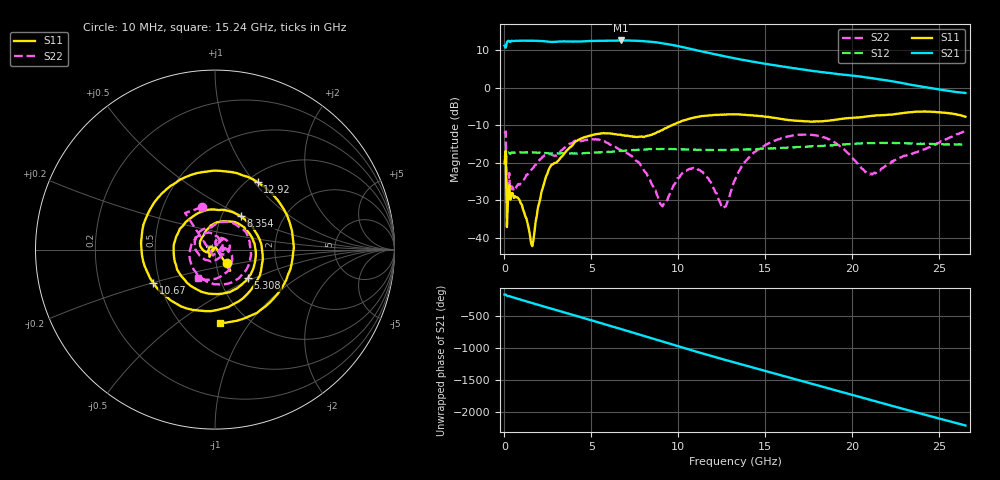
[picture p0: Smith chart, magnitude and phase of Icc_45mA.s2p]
!Keysight Technologies,N5245A,MY52451697,A.10.60.06
!Date: Thursday, May 06, 2021 15:05:53
!Correction: S11(Full 2 Port(1,4))
!S41(Full 2 Port(1,4))
!S14(Full 2 Port(1,4))
!S44(Full 2 Port(1,4))
!S2P File: Measurements: S11, S41, S14, S44:
# Hz S  dB  R 50
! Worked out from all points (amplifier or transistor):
!   401 points, 10 MHz to 26.5 GHz, reference 50 ohm
!   highest |S21| = 12.7 dB at 6.699 GHz (marker M1)
!   |S21| within 3 dB of that: start of sweep to 11.42 GHz
!   unconditionally stable (mu >= 1): start of sweep to end of sweep
!   at 4.381 GHz: K = 1.13, MAG = 12.7 dB, |S12| = -17.4 dB
!   at 13.26 GHz: K = 1.24, MAG = 9.2 dB, |S12| = -16.5 dB
!   at 26.5 GHz: K = 2.53, MAG = 0.0 dB, |S12| = -15.0 dB
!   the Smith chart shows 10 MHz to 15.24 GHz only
!   S11 on the Smith chart (normalised r, x): 10 MHz: 1.13, -0.17; 5.308 GHz: 1.37, -0.46; 8.354 GHz: 1.23, +0.48; 10.67 GHz: 0.46, -0.20; 12.92 GHz: 1.11, +1.04; 15.24 GHz: 0.75, -0.73
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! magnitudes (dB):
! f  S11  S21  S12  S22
! 10 MHz  -20.1  11.3  -18.0  -12.1
! 274.9 MHz  -25.9  12.5  -17.4  -22.7
! 870.9 MHz  -29.9  12.6  -17.2  -25.8
! 1.599 GHz  -42.2  12.6  -17.2  -21.6
! 2.063 GHz  -29.4  12.5  -17.2  -18.9
! 2.593 GHz  -21.3  12.3  -17.5  -17.6
! 4.447 GHz  -13.4  12.4  -17.4  -14.1
! 5.308 GHz  -12.3  12.6  -17.2  -13.7
! 6.699 GHz  -12.5  12.7  -16.8  -16.6
! 8.354 GHz  -12.6  12.4  -16.3  -24.3
! 8.884 GHz  -11.6  12.1  -16.3  -30.0
! 9.215 GHz  -10.8  11.8  -16.3  -30.9
! 10.67 GHz  -8.2  10.5  -16.5  -21.5
! 11.6 GHz  -7.4  9.5  -16.5  -23.4
! 12.59 GHz  -7.1  8.5  -16.5  -31.9
! 12.92 GHz  -7.0  8.2  -16.5  -29.1
! 13.26 GHz  -7.0  7.9  -16.5  -24.5
! 15.24 GHz  -7.8  6.3  -16.1  -14.7
! 17.69 GHz  -9.0  4.6  -15.5  -12.5
! 20.87 GHz  -7.6  2.8  -14.7  -22.7
! 22.13 GHz  -7.1  1.9  -14.7  -20.1
! 26.5 GHz  -7.7  -1.3  -15.0  -11.5
